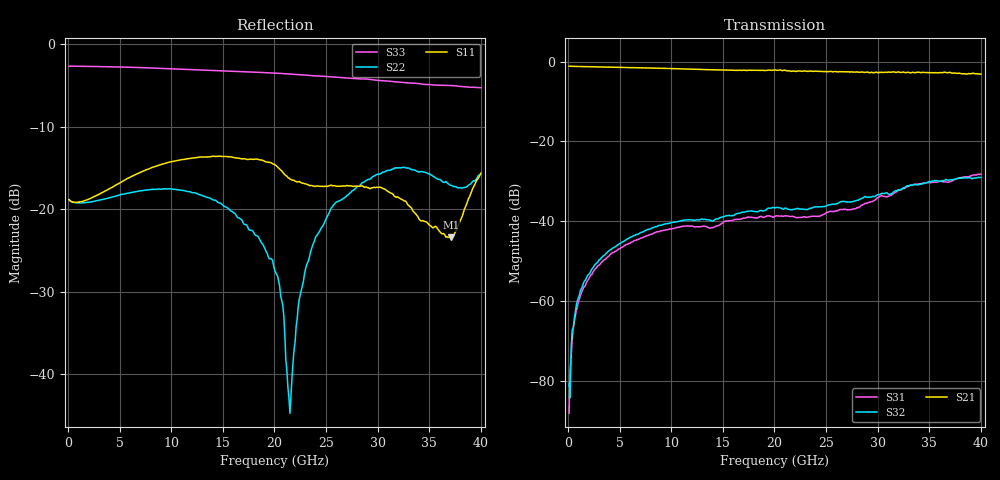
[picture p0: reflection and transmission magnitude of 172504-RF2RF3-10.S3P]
!  3-Port S-parameters saved by WinCal
! VAR MeasName=S-Parameters (CALIBRATED_DATA) read from VNA (N5245A)
! VAR MeasDate=2017-3-15 11:03:45
! VAR NAME=172504-RF2RF3-10
! VAR FILENAME=172504-RF2RF3-10.S3P
! VAR DATE=2017-3-15 11:03:46
! VAR PHYS_PORTS=1,2,3
# Hz S DB R 50
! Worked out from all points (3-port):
!   400 points, 100 MHz to 40 GHz, reference 50 ohm
!   strongest paths, dB at 100 MHz, 10.1 GHz, 20.1 GHz, 30.1 GHz, 40 GHz:
!     S21: -1.1, -1.7, -2.0, -2.7, -3.1
!     S32: -80.8, -40.3, -36.6, -33.3, -29.0
!     S31: -88.2, -41.9, -38.7, -34.0, -28.2
!   lowest |S11| = -23.4 dB at 37.1 GHz (marker M1), VSWR 1.14, Z = 49.1 + j6.64 ohm
!   |S11| at or under -10 dB: start of sweep to end of sweep
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1e8  -18.85 -2.9  -1.10 -0.8  -82.05 157.0
     -1.10 -0.8  -18.85 -2.6  -80.83 120.3
     -88.23 130.5  -80.82 163.7  -2.64 179.8
4e8  -19.11 -8.3  -1.14 -2.8  -70.42 106.9
     -1.14 -2.8  -19.12 -7.5  -68.08 110.8
     -69.69 118.4  -67.25 94.7  -2.64 179.2
1.2e9  -19.10 -21.3  -1.19 -7.8  -58.85 88.9
       -1.19 -7.8  -19.25 -18.6  -57.55 88.7
       -58.59 91.7  -57.31 90.1  -2.65 177.5
3.9e9  -17.58 -58.2  -1.33 -24.1  -48.92 67.5
       -1.33 -24.2  -18.65 -53.2  -47.58 65.4
       -48.90 67.5  -47.55 65.0  -2.71 172.0
2.01e10  -14.63 -153.5  -2.10 -117.9  -38.42 -16.9
         -2.03 -118.2  -27.64 -161.8  -36.19 -30.0
         -38.71 -15.9  -36.63 -29.8  -3.47 138.5
2.15e10  -16.33 -154.4  -2.32 -126.8  -38.62 -26.6
         -2.31 -127.5  -44.77 -91.3  -36.84 -39.8
         -38.81 -24.7  -37.09 -36.4  -3.60 135.0
2.24e10  -16.62 -151.9  -2.55 -131.6  -39.08 -28.8
         -2.30 -131.7  -30.92 -43.4  -36.67 -42.7
         -39.06 -26.5  -36.99 -40.5  -3.67 132.8
2.55e10  -17.07 -147.3  -2.58 -149.5  -37.51 -33.5
         -2.41 -149.8  -19.85 -51.7  -35.55 -50.4
         -37.53 -31.7  -35.78 -48.6  -3.93 125.1
3.71e10  -23.42 93.8  -2.92 138.2  -29.88 -108.6
         -2.74 137.0  -17.09 -91.1  -29.39 -124.7
         -30.04 -106.0  -29.59 -121.4  -4.98 92.4
4e10  -15.63 33.9  -3.09 118.7  -27.97 -133.2
      -3.07 117.3  -15.70 -72.6  -28.84 -146.7
      -28.18 -131.3  -29.01 -145.5  -5.25 82.6
